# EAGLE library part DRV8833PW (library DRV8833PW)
Motor / Motion / Ignition Controllers & Drivers DRV8833 EVAL MOD Source: Datasheet
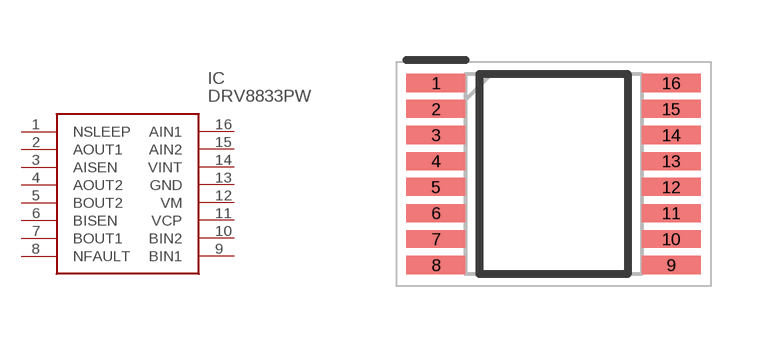
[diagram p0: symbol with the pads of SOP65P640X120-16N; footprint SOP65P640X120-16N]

Designator prefix IC

## DRV8833PW (Description: Motor / Motion / Ignition Controllers & Drivers DRV8833 EVAL MOD; Height: 1.2mm; Manufacturer_Name: Texas Instruments; Manufacturer_Part_Number: DRV8833PW; Mouser_Part_Number: 595-DRV8833PW; Mouser_Price-Stock: https://www.mouser.co.uk/ProductDetail/Texas-Instruments/DRV8833PW?qs=biyDIajrTn6dSTURhvWZBQ%3D%3D)  [SOP65P640X120-16N]
1  NSLEEP
2  AOUT1
3  AISEN
4  AOUT2
5  BOUT2
6  BISEN
7  BOUT1
8  NFAULT
9  BIN1
10  BIN2
11  VCP
12  VM
13  GND
14  VINT
15  AIN2
16  AIN1

## Footprint SOP65P640X120-16N (pad centres in mm)
PW
smd 1.475 x 0.45: 1 -2.938,2.275; 2 -2.938,1.625; 3 -2.938,0.975; 4 -2.938,0.325; 5 -2.938,-0.325; 6 -2.938,-0.975; 7 -2.938,-1.625; 8 -2.938,-2.275; 9 2.938,-2.275; 10 2.938,-1.625; 11 2.938,-0.975; 12 2.938,-0.325; 13 2.938,0.325; 14 2.938,0.975; 15 2.938,1.625; 16 2.938,2.275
